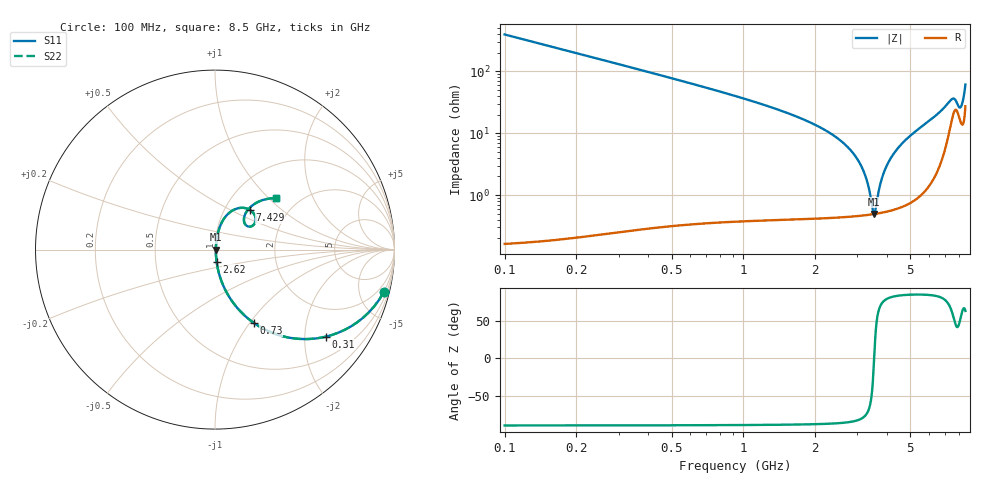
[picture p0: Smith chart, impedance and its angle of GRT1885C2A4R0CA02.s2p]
!Murata Part Number: GRT1885C2A4R0CA02
!These Parameters are Measured in Series Mode Connection
!Data Generated on Jun 19, 2026
!  o--ll--o
!Port1  Port2
!  o------o
!Operation Temp=25[degC], DC Bias Voltage=0[V]
!Freq. Start=100[MHz] Stop=9[GHz] 401[Steps]
# Hz S RI R 50
!Freq.(Hz) S11(Real) S11(Imag) S21(Real) S21(Imag) S12(Real) S12(Imag) S22(Real) S22(Imag)
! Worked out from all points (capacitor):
!   401 points, 100 MHz to 8.5 GHz, reference 50 ohm
!   read as one part in series: C = 4 pF near 142 MHz
!   lowest |Z| = 492 mohm at 3.523 GHz (marker M1)
!   series resonance near 3.526 GHz, so ESL is about 510 pH
!   S11 on the Smith chart (normalised r, x): 100 MHz: 1.00, -7.95; 310 MHz: 1.01, -2.55; 730 MHz: 1.01, -1.04; 2.62 GHz: 1.01, -0.14; 7.429 GHz: 1.31, +0.63; 8.5 GHz: 1.55, +1.10
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1e8  0.9404 -0.2365  0.0596 0.2365  0.0596 0.2365  0.9404 -0.2365
2.05e8  0.7887 -0.4077  0.2113 0.4077  0.2113 0.4077  0.7887 -0.4077
3.1e8  0.6181 -0.4849  0.3819 0.4849  0.3819 0.4849  0.6181 -0.4849
4.99e8  0.3793 -0.4832  0.6207 0.4832  0.6207 0.4832  0.3793 -0.4832
7.3e8  0.2155 -0.4078  0.7845 0.4078  0.7845 0.4078  0.2155 -0.4078
1.507e9  0.0484 -0.2057  0.9516 0.2057  0.9516 0.2057  0.0484 -0.2057
2.62e9  0.00912 -0.0687  0.9909 0.0687  0.9909 0.0687  0.00912 -0.0687
2.914e9  0.00646 -0.0441  0.9935 0.0441  0.9935 0.0441  0.00646 -0.0441
3.25e9  0.00506 -0.019  0.9949 0.019  0.9949 0.019  0.00506 -0.019
3.523e9  0.0049 -0.000193  0.9951 0.000193  0.9951 0.000193  0.0049 -0.000193
3.565e9  0.00494 0.00259  0.9951 -0.00259  0.9951 -0.00259  0.00494 0.00259
3.733e9  0.00527 0.0135  0.9947 -0.0135  0.9947 -0.0135  0.00527 0.0135
3.859e9  0.00567 0.0215  0.9943 -0.0215  0.9943 -0.0215  0.00567 0.0215
4.3e9  0.00813 0.0482  0.9919 -0.0482  0.9919 -0.0482  0.00813 0.0482
4.867e9  0.0137 0.0814  0.9863 -0.0814  0.9863 -0.0814  0.0137 0.0814
5.707e9  0.0289 0.1318  0.9711 -0.1318  0.9711 -0.1318  0.0289 0.1318
7.114e9  0.128 0.2302  0.872 -0.2302  0.872 -0.2302  0.128 0.2302
7.429e9  0.1936 0.2217  0.8064 -0.2217  0.8064 -0.2217  0.1936 0.2217
7.702e9  0.2259 0.1607  0.7741 -0.1607  0.7741 -0.1607  0.2259 0.1607
8.08e9  0.1649 0.147  0.8351 -0.147  0.8351 -0.147  0.1649 0.147
8.311e9  0.1859 0.225  0.8141 -0.225  0.8141 -0.225  0.1859 0.225
8.5e9  0.3388 0.2862  0.6612 -0.2862  0.6612 -0.2862  0.3388 0.2862
